{attribute 'no_assign'}
FUNCTION_BLOCK FB_DO_IED_MUnn_LLN0_NamPlt EXTENDS FB_AcsiCommonDataClass
VAR_INPUT
	vendor: FB_AcsiDATypeVisString255 := (Fc:=ACSI_FC_DC, sValue:='BECKHOFF', bLinkResult:=THIS^.AddDataToContainer(ipData:=vendor));
	swRev: FB_AcsiDATypeVisString255 := (Fc:=ACSI_FC_DC, sValue:='1.0.0', bLinkResult:=THIS^.AddDataToContainer(ipData:=swRev));
	ldNs: FB_AcsiDATypeVisString255 := (Fc:=ACSI_FC_EX, sValue:='IEC 61850-7-4:2007', bLinkResult:=THIS^.AddDataToContainer(ipData:=ldNs));
END_VAR
VAR
END_VAR

END_FUNCTION_BLOCK
